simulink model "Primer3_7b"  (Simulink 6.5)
settings: Solver=ode23t  StartTime=0.0  StopTime=5  RelTol=1e-3
undefined symbols (not defined in the file or in its folder): blocks, Continuous, powergui, ZData
libraries: powerlib x3, powerlib_extras x2

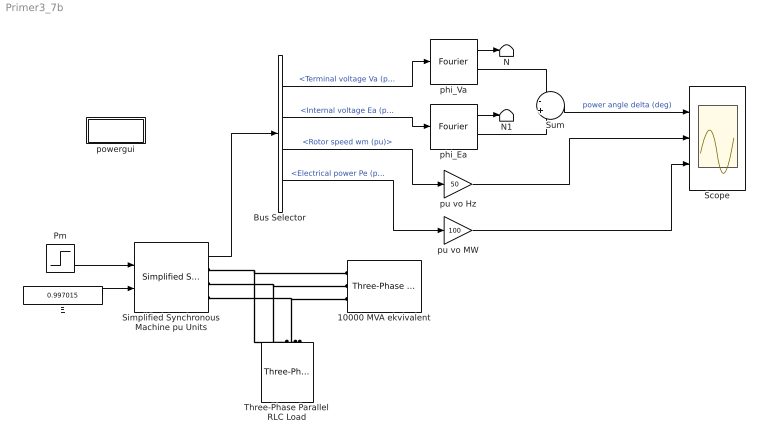
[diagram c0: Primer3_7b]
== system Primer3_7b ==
  10000 MVA ekvivalent : powerlib/Electrical Sources/Three-Phase Source  Orientation=left  DialogController=PMDialogs.PMDefaultMaskDlg  SystemSampleTime=-1  Voltage=10.5e3  PhaseAngle=0  Frequency=50  InternalConnection=Yg  SpecifyImpedance=on  Resistance=5.55  Inductance=0.221  ShortCircuitLevel=10000e6  BaseVoltage=10.5e3  XRratio=10
  Bus Selector : BusSelector  OutputSignals=Terminal voltage Va (pu),Internal voltage Ea (pu),Rotor speed wm (pu),Electrical power Pe (pu)
  E : Constant  Value=0.997015  OutDataType=sfix(16)  ConRadixGroup=Use specified scaling  OutScaling=2^0  SampleTime=inf  FramePeriod=inf
  N : Terminator
  N1 : Terminator
  Pm : Step  Time=0.5  Before=0.5  After=0.6  SampleTime=0
  Scope : Scope  NumInputPorts=3
  Simplified Synchronous Machine pu Units : powerlib/Machines/Simplified Synchronous Machine pu Units  DialogController=PMDialogs.PMDefaultMaskDlg  SystemSampleTime=-1  ConnectionType=3-wire Y  NominalParameters=[100e6 10.5e3 50]  Mechanical=[6 20 1]  InternalRL="[0  0.3]"  InitialConditions=[0 8.93644 0.502277 0.502277 0.502277 5.74164 -114.258 125.742]  Units=0  LoadFlowParameters=[1 50000000 0 0 0]
  Sum : Sum  Inputs=-+
  Three-Phase Parallel RLC Load : powerlib/Elements/Three-Phase Parallel RLC Load  Orientation=down  DialogController=PMDialogs.PMDefaultMaskDlg  PhysicalDomain=powersysdomain  SubClassName=unknown  LeftPortType=p1  RightPortType=p1  LConnTagsString=A|B|C  Configuration=Y (grounded)  NominalVoltage=10.5e3  NominalFrequency=50  ActivePower=1e6  InductivePower=0  CapacitivePower=0  Measurements=None
  phi_Ea : powerlib_extras/Measurements/Fourier  DialogController=PMDialogs.PMDefaultMaskDlg  SystemSampleTime=-1  f1=50  n=1
  phi_Va : powerlib_extras/Measurements/Fourier  DialogController=PMDialogs.PMDefaultMaskDlg  SystemSampleTime=-1  f1=50  n=1
  powergui : Subsystem  AncestorBlock=powerlib/powergui  InitFcn=powergui( 'InitFcn_Callback' , gcb , 0 , [ ] );  mask(PSB option menu block){SimulationMode=Continuous, SampleTime=50e-6, echomessages=off, RestoreLinks=warning, x0status=blocks, Frange=[0:2:500], Ylog=off, Xlog=on, ShowGrid=off, save=off, variable=ZData, structure=, ZoomFFT=on, StartTime=0.0, cycles=1, DisplayStyle=1, fundamental=60, FreqAxis=off, MaxFrequency=1000, frequencyindice=50, frequencyindicesteady=1, RmsSteady=1, display=off, Ts=0, frequency=60, methode=off, HookPort=off, Interpol=off}
      mask prompts: SimulationMode "Simulation mode"; SampleTime "Sample time Ts (when simulation mode is Discrete) (s)"; echomessages "Echo  Messages"; RestoreLinks "Restore disabled links"; x0status "Initial electrical states status"; Frange "Impedance tool: Frequency Range"; Ylog "Impedance tool: Log impedance"; Xlog "Impedance tool: log Frequency"; ShowGrid "Impedance tool: grid"; save "Impedance tool: Save Data To Workspace"; variable "Impedance tool: Variable Name"; structure "Structure Name (PSBFFTSCOPE)"; ZoomFFT "ZoomFFT (PSBFFTSCOPE)"; StartTime "Start Time (PSBFFTSCOPE)"; cycles "Cycles (PSBFFTSCOPE)"; DisplayStyle "Display style (PSBFFTSCOPE)"; fundamental "Fundamental (PSBFFTSCOPE)"; FreqAxis "Frequency Axis (PSBFFTSCOPE)"; MaxFrequency "Max Frequency (PSBFFTSCOPE)"; frequencyindice "Load flow frequency (Hz)"; frequencyindicesteady "Frequency indice (STEADYSTATE)"; RmsSteady "RMS display (STEADYSTATE)"; display "Display Results"; Ts "OBSOLETE 1"; frequency "Phasor frequency (Hz)"; methode "Phasor simulation"; HookPort "Hook port"; Interpol "Interpolate"
      mask init:
      | powerlibroot = which('powersysdomain');
      | PSBroot = powerlibroot(1:end-16);
      | %
      | switch SimulationMode
      | 	case 1
      | 		message=sprintf('Continuous');
      | 	case 2
      |         SampleTimeeval=evalin('base',SampleTime,'NaN');
      |         if isnan(SampleTimeeval)
      |             message=sprintf('Warning !!,\nUndefined sample time');
      |         else
      |             message=sprintf('Discrete,\nTs = %.4g s.',SampleTimeeval);
      |         end
      | 	case 3
      | 		message=sprintf('Phasors');
      | end
      | if strcmp(bdroot,'powerlib')
      |   message='powergui';
      | end
      | power_initmask();
  pu vo Hz : Gain  Gain=50
  pu vo MW : Gain  Gain=100
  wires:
  E/1 -> Simplified Synchronous Machine pu Units/2
  Pm/1 -> Simplified Synchronous Machine pu Units/1
  phi_Va/2 -> Sum/1
  phi_Ea/2 -> Sum/2
  Sum/1 -> Scope/1  "power angle delta (deg)"
  phi_Va/1 -> N/1
  phi_Ea/1 -> N1/1
  Bus Selector/1 -> phi_Va/1  "<Terminal voltage Va (pu)>"
  Bus Selector/2 -> phi_Ea/1  "<Internal voltage Ea (pu)>"
  Simplified Synchronous Machine pu Units/1 -> Bus Selector/1
  Bus Selector/3 -> pu vo Hz/1  "<Rotor speed wm (pu)>"
  pu vo Hz/1 -> Scope/2
  Bus Selector/4 -> pu vo MW/1  "<Electrical power Pe (pu)>"
  pu vo MW/1 -> Scope/3
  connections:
  Simplified Synchronous Machine pu Units/RConn3 -- 10000 MVA ekvivalent/RConn3 -- Three-Phase Parallel RLC Load/LConn3
  Simplified Synchronous Machine pu Units/RConn2 -- 10000 MVA ekvivalent/RConn2 -- Three-Phase Parallel RLC Load/LConn2
  Simplified Synchronous Machine pu Units/RConn1 -- 10000 MVA ekvivalent/RConn1 -- Three-Phase Parallel RLC Load/LConn1

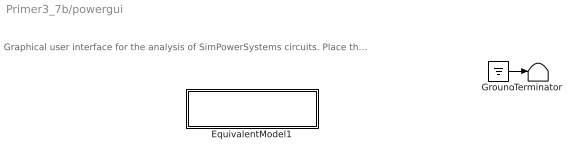
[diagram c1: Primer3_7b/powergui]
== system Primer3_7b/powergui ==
  note: Graphical user interface for the analysis of SimPowerSystems circuits. Place the Powergui block in the top-level of your model and double-click on it to open the GUI.
  EquivalentModel1 : Subsystem
  Ground : Ground
  Terminator : Terminator
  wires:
  Ground/1 -> Terminator/1

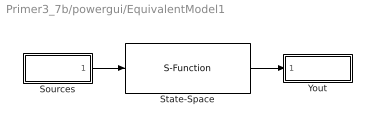
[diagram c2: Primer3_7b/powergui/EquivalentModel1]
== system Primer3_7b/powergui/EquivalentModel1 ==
  Sources : Subsystem
  State-Space : S-Function  FunctionName=sfun_spssw_contc  Parameters=A, B, C, D, x0
  Yout : Subsystem
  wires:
  State-Space/1 -> Yout/1(v,i)
  Sources/1(u) -> State-Space/1

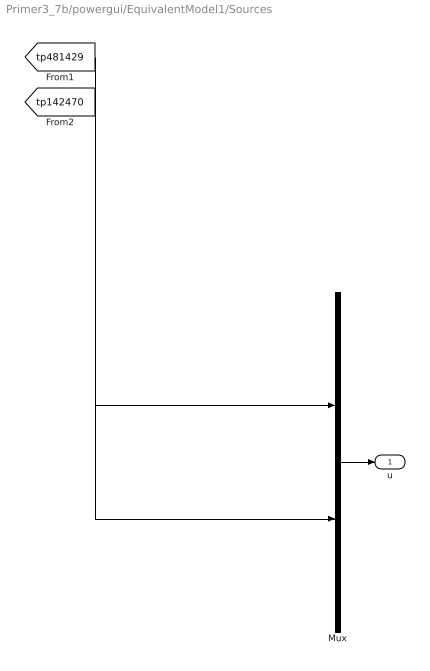
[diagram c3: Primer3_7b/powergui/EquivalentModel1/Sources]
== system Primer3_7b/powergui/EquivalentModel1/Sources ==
  Mux : Mux  Inputs=[2 3]
  u : Outport
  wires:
  Mux/1 -> u/1
  [tp481429] -> Mux/1
  [tp142470] -> Mux/2

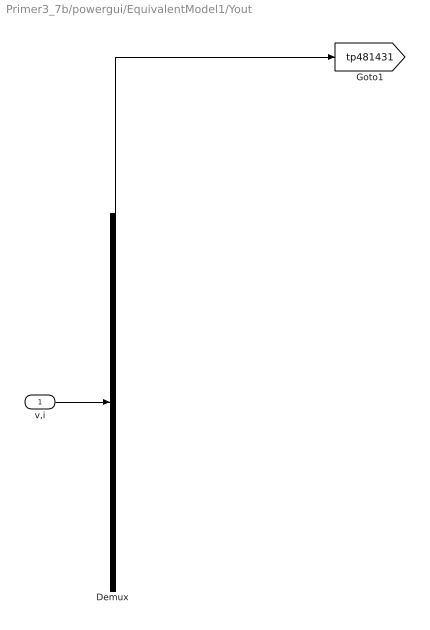
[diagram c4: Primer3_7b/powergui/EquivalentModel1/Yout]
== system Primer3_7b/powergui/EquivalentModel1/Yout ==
  v,i : Inport
  Demux : Demux  Outputs=1
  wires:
  v,i/1 -> Demux/1
  Demux/1 -> [tp481431]
